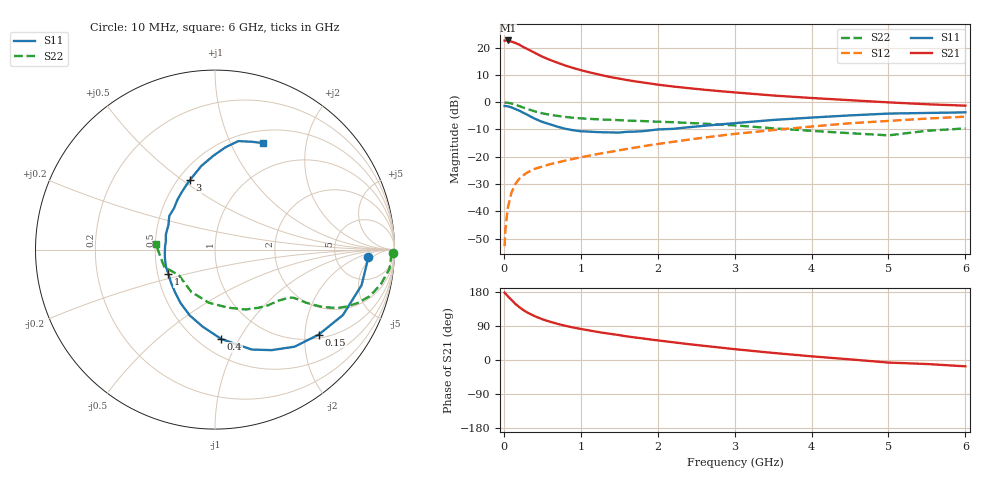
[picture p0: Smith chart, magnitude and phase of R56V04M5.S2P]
! SIEMENS Small Signal Semiconductors
! BFR183
! Si NPN RF Bipolar Junction Transistor in SOT23
! VCE = 6 V  IC = 4.5 mA
! Common Emitter S-Parameters:  May  1996
# GHz  S  MA  R  50
!  f  S11  S21  S12  S22
! GHz  MAG  ANG  MAG  ANG  MAG  ANG  MAG  ANG
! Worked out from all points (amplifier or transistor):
!   36 points, 10 MHz to 6 GHz, reference 50 ohm
!   highest |S21| = 22.6 dB at 50 MHz (marker M1)
!   |S21| within 3 dB of that: start of sweep to 295 MHz
!   unconditionally stable (mu >= 1): 1.122 GHz to 2.686 GHz
!   at 250 MHz: K = 0.39, MSG = 23.6 dB, |S12| = -26.8 dB
!   at 1.4 GHz: K = 1.06, MAG = 12.2 dB, |S12| = -18.1 dB
!   at 6 GHz: K = 0.88, MSG = 2.0 dB, |S12| = -5.3 dB
!   S11 on the Smith chart (normalised r, x): 10 MHz: 11, -4; 150 MHz: 1.10, -2.36; 400 MHz: 0.64, -0.84; 1 GHz: 0.57, -0.17; 3 GHz: 0.57, +0.54; 6 GHz: 0.65, +1.33
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0.01  0.8525 -2.9  13.44 177.8  0.0023 85.8  0.9903 -1.2
0.02  0.8496 -5.4  13.44 175.3  0.0046 90.3  0.982 -2.4
0.05  0.8402 -13.7  13.51 168.8  0.0113 83.9  0.9779 -6.3
0.1  0.8006 -27.1  12.88 158.5  0.0223 75.6  0.9437 -11.9
0.15  0.7472 -39.3  12.19 148.0  0.0317 70.2  0.8994 -16.8
0.2  0.6998 -50.6  11.34 139.7  0.0394 65.8  0.8492 -20.5
0.25  0.643 -60.6  10.31 132.3  0.0455 62.0  0.7988 -23.4
0.3  0.5933 -69.8  9.487 125.9  0.0509 59.9  0.756 -25.5
0.4  0.4991 -86.0  8.053 115.8  0.0599 56.7  0.6791 -28.1
0.5  0.4352 -99.0  6.812 107.5  0.0662 55.0  0.6236 -29.4
0.6  0.3931 -110.9  5.948 101.0  0.073 54.3  0.5879 -30.2
0.8  0.3253 -133.3  4.688 90.2  0.0851 54.8  0.5369 -31.0
1  0.2933 -152.2  3.866 81.9  0.0974 56.1  0.506 -31.9
1.1  0.2894 -160.9  3.558 78.4  0.1042 56.8  0.4957 -32.7
1.3  0.2805 -176.1  3.058 71.5  0.1177 57.5  0.4801 -34.2
1.6  0.2863 163.0  2.543 62.3  0.1391 57.8  0.4613 -37.5
2.2  0.3248 134.6  1.937 46.8  0.188 56.8  0.4299 -46.0
3  0.4125 109.7  1.511 28.6  0.2619 51.5  0.3758 -62.7
3.5  0.4721 99.3  1.325 18.7  0.3083 46.3  0.3321 -77.1
4.5  0.5727 84.2  1.087 1.7  0.4109 34.9  0.2702 -119.3
5.5  0.6345 71.3  0.916 -10.6  0.5009 22.5  0.2991 -161.4
6  0.6507 65.8  0.862 -16.7  0.5424 14.4  0.3308 174.9
